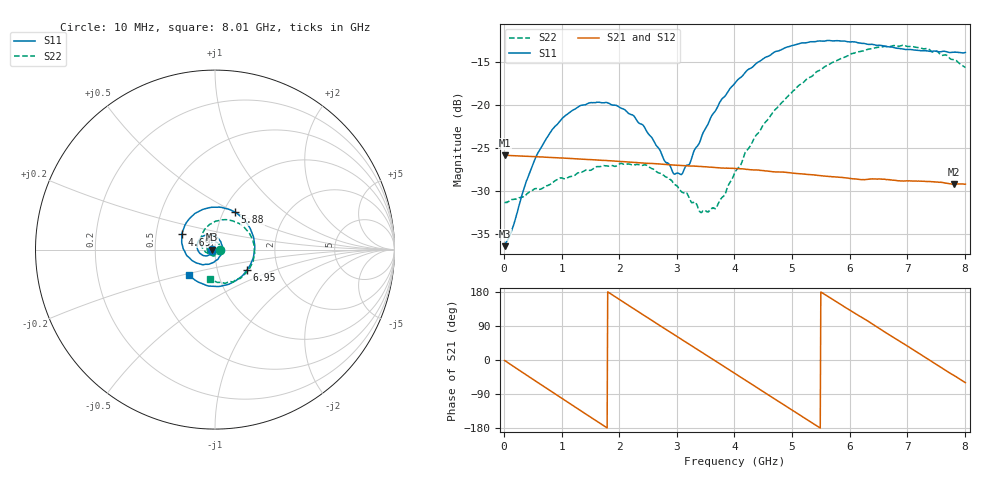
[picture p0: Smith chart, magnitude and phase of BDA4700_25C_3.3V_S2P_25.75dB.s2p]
!Agilent Technologies,E5071B,MY42404982,A.09.10
!Date: Mon Oct 20 18:13:53 2025
!Data & Calibration Information:
!Freq	S11:SOLT2(ON)	S21:SOLT2(ON)	S12:SOLT2(ON)	S22:SOLT2(ON)
# Hz S RI R 50
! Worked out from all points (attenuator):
!   801 points, 10 MHz to 8.01 GHz, reference 50 ohm
!   highest |S21| = -25.81 dB at 10 MHz (marker M1); lowest = -29.2 dB at 7.81 GHz (marker M2)
!   lowest |S11| = -36.4 dB at 10 MHz (marker M3), VSWR 1.03, Z = 48.5 - j0.119 ohm
!   |S11| at or under -10 dB: start of sweep to end of sweep
!   |S22| runs from -32.5 to -13.0 dB; largest |S21 - S12| = 0.00061
!   S11 on the Smith chart (normalised r, x): 10 MHz: 0.97, -0.00; 4.69 GHz: 0.68, +0.12; 5.88 GHz: 1.13, +0.50; 6.95 GHz: 1.39, -0.33; 8.01 GHz: 0.72, -0.21
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1e7  -0.0151 -0.00123  0.0512 -0.00109  0.0512 -0.00114  0.0271 -0.000784
6e8  -0.0411 -0.0344  0.0244 -0.0437  0.0244 -0.0437  0.0132 -0.0296
1.01e9  -0.0802 -0.0245  -0.0101 -0.0482  -0.0101 -0.0482  -0.0152 -0.0345
1.35e9  -0.0996 0.00863  -0.0347 -0.0339  -0.0347 -0.034  -0.0364 -0.0183
2.08e9  -0.0476 0.082  -0.0415 0.0219  -0.0415 0.0219  -0.0302 0.0337
2.42e9  0.00117 0.076  -0.0222 0.0403  -0.0222 0.0404  -0.00525 0.0444
2.68e9  0.0299 0.0478  -0.00275 0.0454  -0.00281 0.0454  0.0128 0.0383
2.94e9  0.0394 0.00787  0.0166 0.0417  0.0166 0.0415  0.0253 0.0247
3.08e9  0.0364 -0.0155  0.0259 0.0363  0.0255 0.0364  0.0282 0.0137
3.41e9  0.00234 -0.0624  0.0406 0.0169  0.0406 0.017  0.0211 -0.0109
3.54e9  -0.0188 -0.0751  0.043 0.00759  0.043 0.00752  0.0141 -0.0195
3.69e9  -0.0485 -0.0819  0.0431 -0.0034  0.0432 -0.00351  0.00159 -0.0252
4.01e9  -0.1164 -0.0674  0.0348 -0.0249  0.0348 -0.0249  -0.0311 -0.0258
4.69e9  -0.1853 0.0842  -0.0085 -0.04  -0.00835 -0.0401  -0.0796 0.0479
5.35e9  -0.0595 0.2264  -0.0382 -0.00954  -0.0381 -0.00973  -0.0161 0.1467
5.88e9  0.1104 0.2088  -0.0303 0.0227  -0.0303 0.0226  0.102 0.1587
6.27e9  0.1984 0.1125  -0.0109 0.0352  -0.0104 0.0352  0.1826 0.1014
6.68e9  0.2166 -0.0285  0.0143 0.0339  0.0144 0.034  0.2193 0.000339
6.95e9  0.1777 -0.1139  0.027 0.0242  0.027 0.024  0.2102 -0.0733
7.42e9  0.0399 -0.2017  0.0358 -0.00217  0.0358 -0.00225  0.1228 -0.1647
7.81e9  -0.0928 -0.1809  0.0263 -0.0226  0.0262 -0.0227  0.0175 -0.1833
8.01e9  -0.1466 -0.14  0.0174 -0.03  0.0176 -0.03  -0.03 -0.1628
